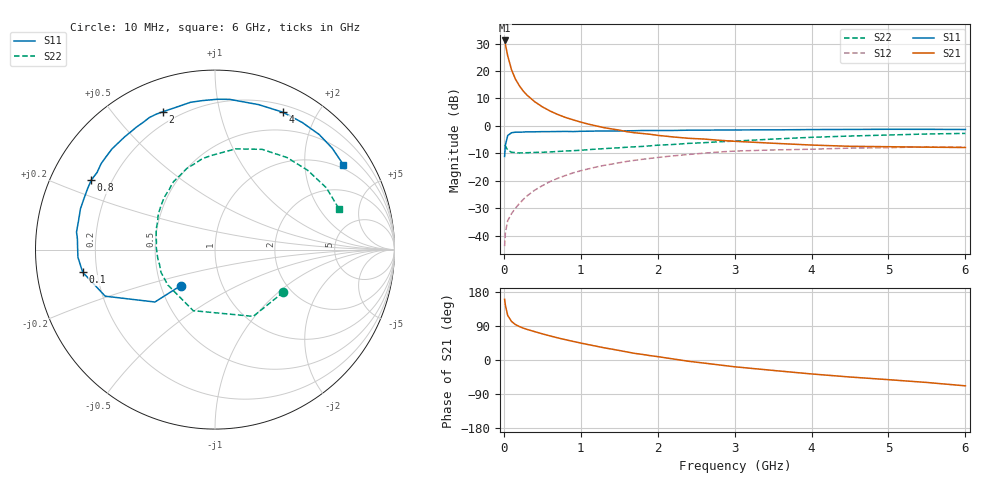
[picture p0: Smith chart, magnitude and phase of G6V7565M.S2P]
! SIEMENS Small Signal Semiconductors
! BFG193
! Si NPN RF Bipolar Junction Transistor in SOT223
! VCE = 0.75 V  IC = 65 mA
! Common Emitter S-Parameters:  August  1996
# GHz  S  MA  R  50
!  f  S11  S21  S12  S22
! GHz  MAG  ANG  MAG  ANG  MAG  ANG  MAG  ANG
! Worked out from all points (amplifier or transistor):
!   36 points, 10 MHz to 6 GHz, reference 50 ohm
!   highest |S21| = 31.1 dB at 10 MHz (marker M1)
!   |S21| within 3 dB of that: start of sweep to 31.86 MHz
!   unconditionally stable (mu >= 1): start of sweep to 19.51 MHz; 118.7 MHz to end of sweep
!   at 250 MHz: K = 1.23, MAG = 17.0 dB, |S12| = -26.9 dB
!   at 1.4 GHz: K = 1.24, MAG = 3.5 dB, |S12| = -14.0 dB
!   at 6 GHz: K = 1.08, MAG = -1.8 dB, |S12| = -7.8 dB
!   S11 on the Smith chart (normalised r, x): 10 MHz: 0.63, -0.28; 100 MHz: 0.15, -0.08; 800 MHz: 0.12, +0.26; 2 GHz: 0.14, +0.68; 4 GHz: 0.28, +1.57; 6 GHz: 0.87, +3.10
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0.01  0.2761 -133.5  35.96 160.2  0.0064 64.7  0.4489 -31.8
0.02  0.4442 -138.9  30.93 144.6  0.0112 58.4  0.4287 -60.2
0.05  0.6644 -157.0  18.9 117.7  0.0186 48.8  0.3613 -109.6
0.1  0.7479 -170.3  10.5 101.7  0.0251 51.2  0.3286 -143.1
0.15  0.7648 -176.8  7.123 93.5  0.0314 55.7  0.3265 -157.3
0.2  0.7656 179.2  5.418 88.5  0.038 59.3  0.32 -164.9
0.25  0.7688 175.6  4.34 84.3  0.0451 61.2  0.3226 -171.3
0.3  0.7777 172.8  3.637 80.9  0.0525 62.4  0.3232 -175.0
0.4  0.7773 167.8  2.755 74.9  0.067 63.1  0.3272 178.0
0.5  0.7833 163.1  2.22 69.0  0.081 62.0  0.3293 172.5
0.6  0.7834 158.8  1.863 63.6  0.0962 61.1  0.3341 168.3
0.8  0.7907 150.7  1.422 53.7  0.1242 57.0  0.3473 160.3
1.1  0.7974 139.6  1.072 40.5  0.1643 50.4  0.3677 149.7
1.6  0.811 122.5  0.781 21.3  0.2246 37.3  0.4073 133.4
2  0.8212 110.6  0.67 8.9  0.2646 26.8  0.4434 121.4
2.2  0.8224 105.0  0.627 2.8  0.2835 21.6  0.4568 115.3
2.8  0.8378 89.0  0.545 -13.0  0.3336 6.1  0.512 97.8
3.5  0.8435 73.2  0.481 -27.5  0.3632 -12.3  0.573 78.4
4  0.8538 63.7  0.446 -36.8  0.3744 -21.8  0.6173 64.8
4.5  0.859 55.5  0.423 -44.9  0.3922 -31.4  0.651 52.0
5.5  0.8636 40.9  0.408 -59.3  0.4149 -52.9  0.7097 29.0
6  0.8574 33.5  0.402 -68.2  0.4095 -65.1  0.7271 18.2
